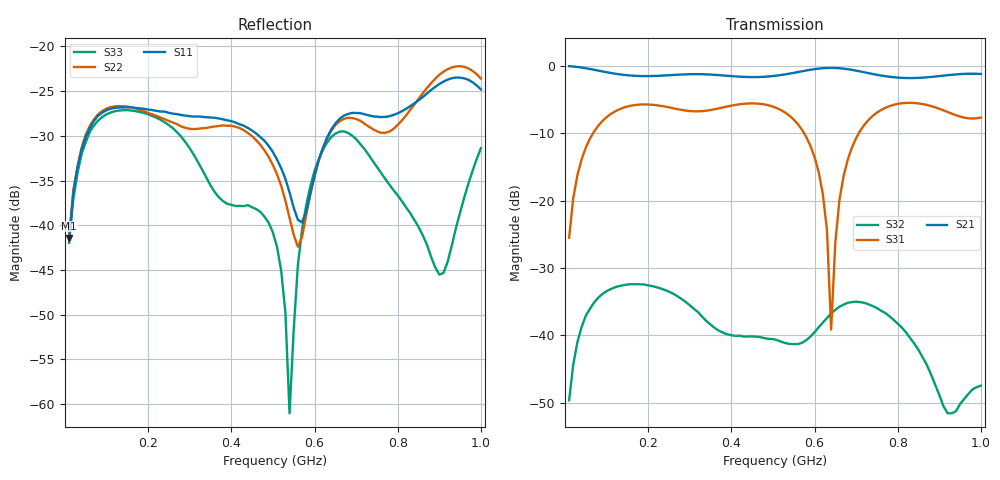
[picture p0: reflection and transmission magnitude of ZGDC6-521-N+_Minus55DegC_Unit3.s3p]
!Created: 04-01-2020 at 16:35:24
!Mini-Circuits
!S3P DATA File Format
!Type: Directional Coupler
!Port 1: (Input); Port 2: (Output); Port 3: (Couple)
!TEST CONDITIONS: Z:50 OHM SYSTEM, INPUT POWER = -10dBm, TEMP:-55°C
!MODEL: ZGDC6-521-N+
!S/N: U3_-55C
# MHZ S DB R 50
!Frequency
!  S11 dB  S11 DEG  S12 dB  S12 DEG  S13 dB  S13 DEG
!  S21 dB  S21 DEG  S22 dB  S22 DEG  S23 dB  S23 DEG
!  S31 dB  S31 DEG  S32 dB  S32 DEG  S33 dB  S33 DEG
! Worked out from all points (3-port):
!   100 points, 10 MHz to 1 GHz, reference 50 ohm
!   strongest paths, dB at 10 MHz, 260 MHz, 510 MHz, 760 MHz, 1 GHz:
!     S21: 0.0, -1.3, -1.4, -1.4, -1.2
!     S31: -25.5, -6.3, -6.3, -6.5, -7.7
!     S32: -49.6, -33.8, -40.7, -36.3, -47.5
!   lowest |S11| = -41.4 dB at 10 MHz (marker M1), VSWR 1.02, Z = 50.3 + j0.797 ohm
!   |S11| at or under -10 dB: start of sweep to end of sweep
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10  -41.43 69.2  -0.04 -7.4  -25.49 83.2
    -0.03 -7.4  -41.62 58.4  -50.08 -105.9
    -25.50 83.1  -49.63 -110.5  -41.96 75.9
130  -26.83 8.3  -1.23 -87.7  -6.45 15.3
     -1.23 -87.7  -26.67 -25.2  -32.67 105.6
     -6.45 15.3  -32.68 105.7  -27.17 2.8
280  -27.68 -16.9  -1.27 -178.5  -6.52 -34.5
     -1.27 -178.5  -28.96 -148.5  -34.59 -46.4
     -6.52 -34.6  -34.59 -46.4  -30.12 -48.2
510  -32.66 -50.4  -1.43 39.2  -6.27 -97.2
     -1.42 39.2  -34.32 -35.9  -40.72 118.5
     -6.27 -97.2  -40.70 118.7  -42.44 -50.7
540  -36.33 -46.5  -1.14 20.9  -7.39 -112.2
     -1.13 20.9  -39.19 -77.6  -41.20 71.1
     -7.40 -112.2  -41.27 71.4  -61.02 -16.5
610  -32.73 29.1  -0.40 -26.0  -15.76 -155.0
     -0.39 -26.1  -32.78 102.9  -38.86 -70.5
     -15.76 -155.0  -38.80 -70.7  -32.63 59.5
640  -29.29 20.6  -0.29 -47.8  -39.18 130.0
     -0.29 -47.8  -29.47 64.7  -36.80 -127.2
     -39.15 130.4  -36.75 -127.5  -30.14 34.0
720  -27.59 -5.3  -0.94 -103.9  -8.72 -39.8
     -0.94 -103.9  -28.64 -33.0  -35.23 107.9
     -8.72 -39.7  -35.17 108.0  -31.47 -18.7
870  -25.27 -12.4  -1.69 167.0  -5.79 -108.0
     -1.69 167.0  -24.67 152.0  -44.36 -58.1
     -5.79 -108.0  -44.38 -58.0  -42.13 -68.5
1000  -24.81 -80.0  -1.18 82.9  -7.65 -127.0
      -1.18 82.9  -23.58 61.6  -47.41 -134.0
      -7.65 -127.0  -47.47 -134.4  -31.39 133.2
